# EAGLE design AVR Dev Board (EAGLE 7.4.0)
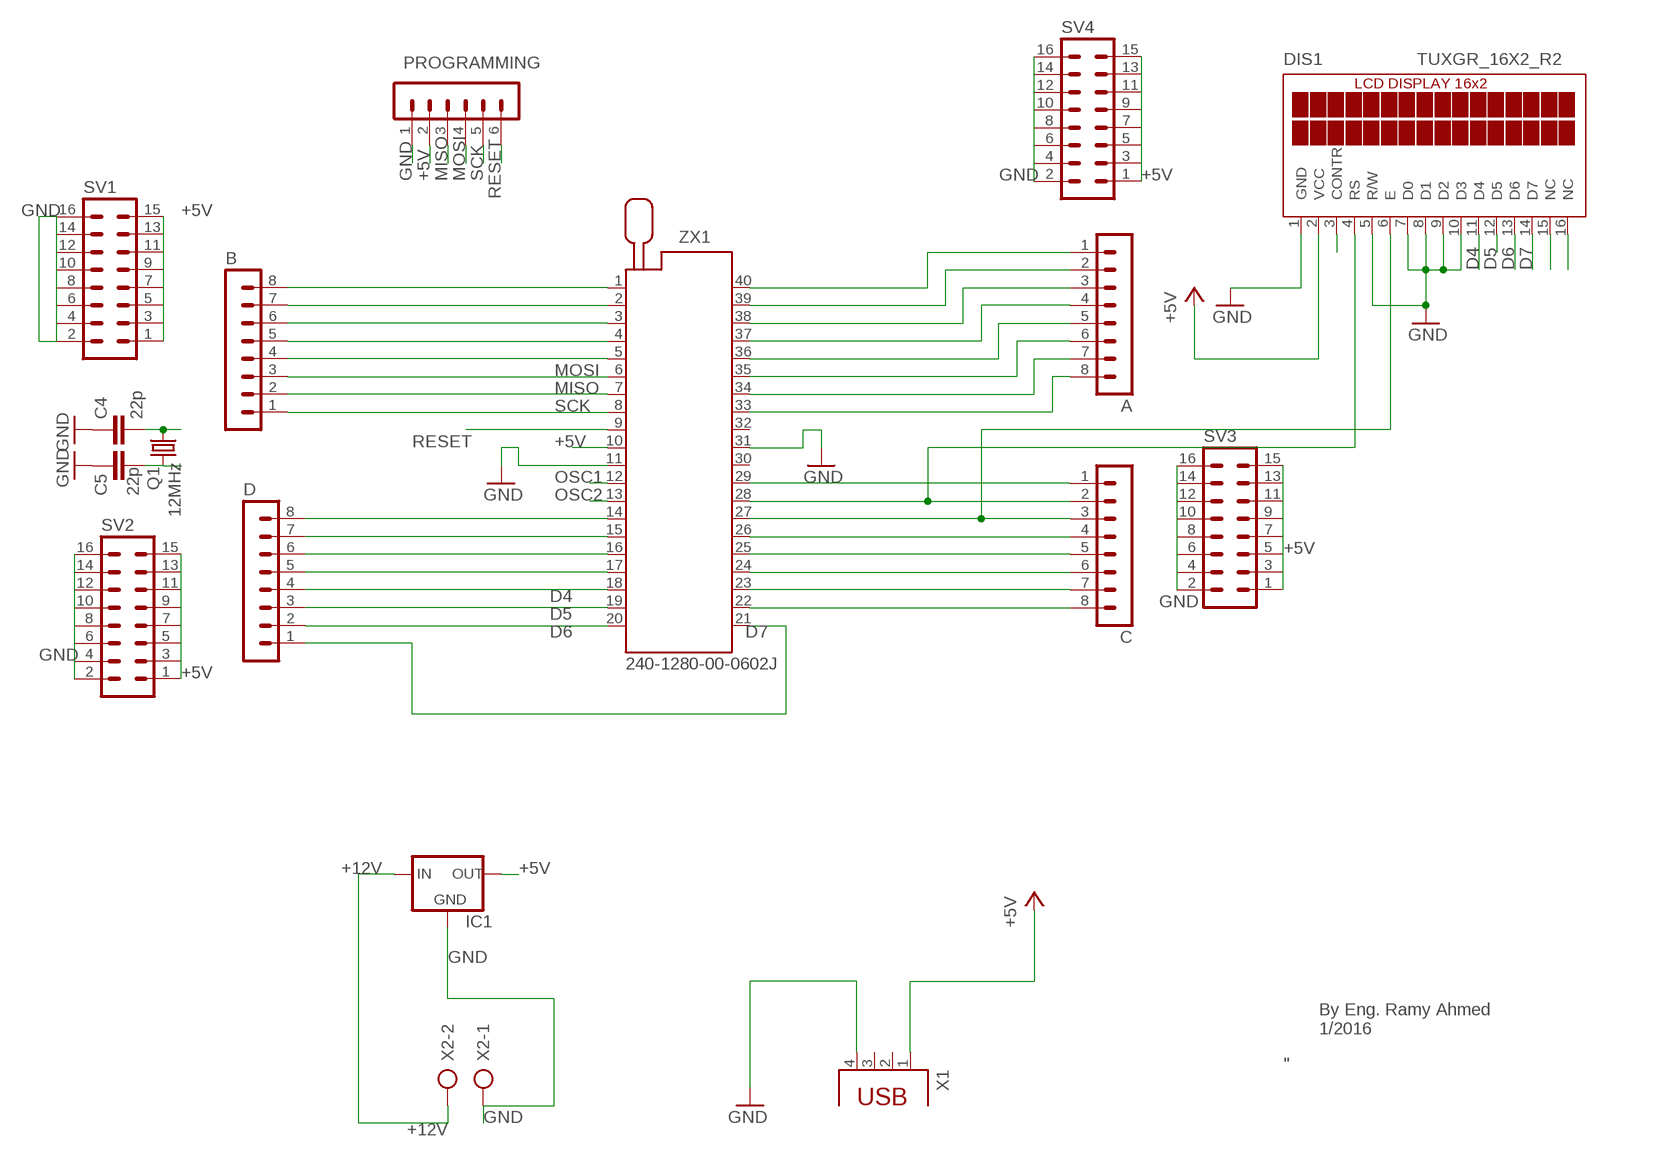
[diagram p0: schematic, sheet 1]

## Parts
A  MA08-1  [MA08-1]
B  MA08-1  [MA08-1]
C  MA08-1  [MA08-1]
C4  22p  C-EU025-024X044  [C025-024X044]
C5  22p  C-EU025-024X044  [C025-024X044]
D  MA08-1  [MA08-1]
DIS1  TUXGR_16X2_R2  [TUXGR_16X2_R2]
IC1  78XXL  [78XXL]
PROGRAMMING  MA06-1  [MA06-1]
Q1  12MHz  CRYTALHC49S  [HC49/S]
SV1  MA08-2  [MA08-2]
SV2  MA08-2  [MA08-2]
SV3  MA08-2  [MA08-2]
SV4  MA08-2  [MA08-2]
X1  PN61729  [PN61729]
X2  AK500/2  [AK500/2]
ZX1  240-1280-00-0602J  [240-1280-00-0602J]

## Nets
+5V: DIS1.2(VCC) IC1.OUT PROGRAMMING.2 SV1.1 SV1.3 SV1.5 SV1.7 SV1.9 SV1.11 SV1.13 SV1.15 SV2.1 SV2.3 SV2.5 SV2.7 SV2.9 SV2.11 SV2.13 SV2.15 SV3.1 SV3.3 SV3.5 SV3.7 SV3.9 SV3.11 SV3.13 SV3.15 SV4.1 SV4.3 SV4.5 SV4.7 SV4.9 SV4.11 SV4.13 SV4.15 X1.1 ZX1.10
+12V: IC1.IN X2.2
D4: D.4 DIS1.11(D4) ZX1.18
D5: D.3 DIS1.12(D5) ZX1.19
D6: D.2 DIS1.13(D6) ZX1.20
D7: D.1 DIS1.14(D7) ZX1.21
GND: C4.1 C5.1 DIS1.1(GND) DIS1.5(R/W) DIS1.7(D0) DIS1.8(D1) DIS1.9(D2) DIS1.10(D3) IC1.GND PROGRAMMING.1 SV1.2 SV1.4 SV1.6 SV1.8 SV1.10 SV1.12 SV1.14 SV1.16 SV2.2 SV2.4 SV2.6 SV2.8 SV2.10 SV2.12 SV2.14 SV2.16 SV3.2 SV3.4 SV3.6 SV3.8 SV3.10 SV3.12 SV3.14 SV3.16 SV4.2 SV4.4 SV4.6 SV4.8 SV4.10 SV4.12 SV4.14 SV4.16 X1.4 X2.1 ZX1.11 ZX1.31
MISO: B.2 PROGRAMMING.3 ZX1.7
MOSI: B.3 PROGRAMMING.4 ZX1.6
N$1: A.6 ZX1.35
N$2: A.1 ZX1.40
N$3: A.2 ZX1.39
N$4: A.3 ZX1.38
N$5: A.4 ZX1.37
N$6: A.5 ZX1.36
N$7: A.8 ZX1.33
N$8: A.7 ZX1.34
N$9: C.8 ZX1.22
N$10: C.7 ZX1.23
N$11: C.6 ZX1.24
N$16: C.5 ZX1.25
N$18: C.4 ZX1.26
N$21: C.1 ZX1.29
N$29: D.5 ZX1.17
N$30: D.6 ZX1.16
N$31: D.7 ZX1.15
N$32: D.8 ZX1.14
N$33: B.8 ZX1.1
N$34: B.7 ZX1.2
N$35: B.6 ZX1.3
N$36: B.5 ZX1.4
N$37: B.4 ZX1.5
N$38: DIS1.3(CONTR)
N$39: C.2 DIS1.4(RS) ZX1.28
N$50: DIS1.15(NC)
N$51: DIS1.16(NC)
N$52: C.3 DIS1.6(E) ZX1.27
OSC1: C4.2 Q1.2 ZX1.12
OSC2: C5.2 Q1.1 ZX1.13
RESET: PROGRAMMING.6 ZX1.9
SCK: B.1 PROGRAMMING.5 ZX1.8
Unconnected: X1.2 X1.3 ZX1.30 ZX1.32

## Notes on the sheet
- By Eng. Ramy Ahmed
  1/2016
- " اللهم انى اعوذ بك من علم لا ينفع "

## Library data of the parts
A B C D = con-lstb:MA08-1: PIN HEADER; OC_FARNELL: unknown; OC_NEWARK: unknown
C4 C5 = rcl:C-EU: CAPACITOR, European symbol
DIS1 = display-lcd:TUXGR_16X2_R2: Tuxgraphics LCD display 16x2 characters reflective, without background light Source: tuxgr_12x2_r2.pdf; OC_FARNELL: unknown; OC_NEWARK: unknown
IC1 = v-reg-2:78XXL: VOLTAGE REGULATOR
PROGRAMMING = con-lstb:MA06-1: PIN HEADER; OC_FARNELL: unknown; OC_NEWARK: unknown
Q1 = crystal:CRYTAL: CRYSTAL
SV1-SV4 = con-lstb:MA08-2: PIN HEADER; OC_FARNELL: unknown; OC_NEWARK: unknown
X1 = con-berg:PN61729: BERG USB connector
X2 = con-ptr500:AK500/2: CONNECTOR; OC_FARNELL: unknown; OC_NEWARK: unknown
ZX1 = con-3m:240-?-00-0602J: Zero Insertion Force Socked Source: http://www.3M.com/ehpd; MF: 3M; MPN: 240-1280-00-0602J; OC_FARNELL: 9897364; OC_NEWARK: 85K7848

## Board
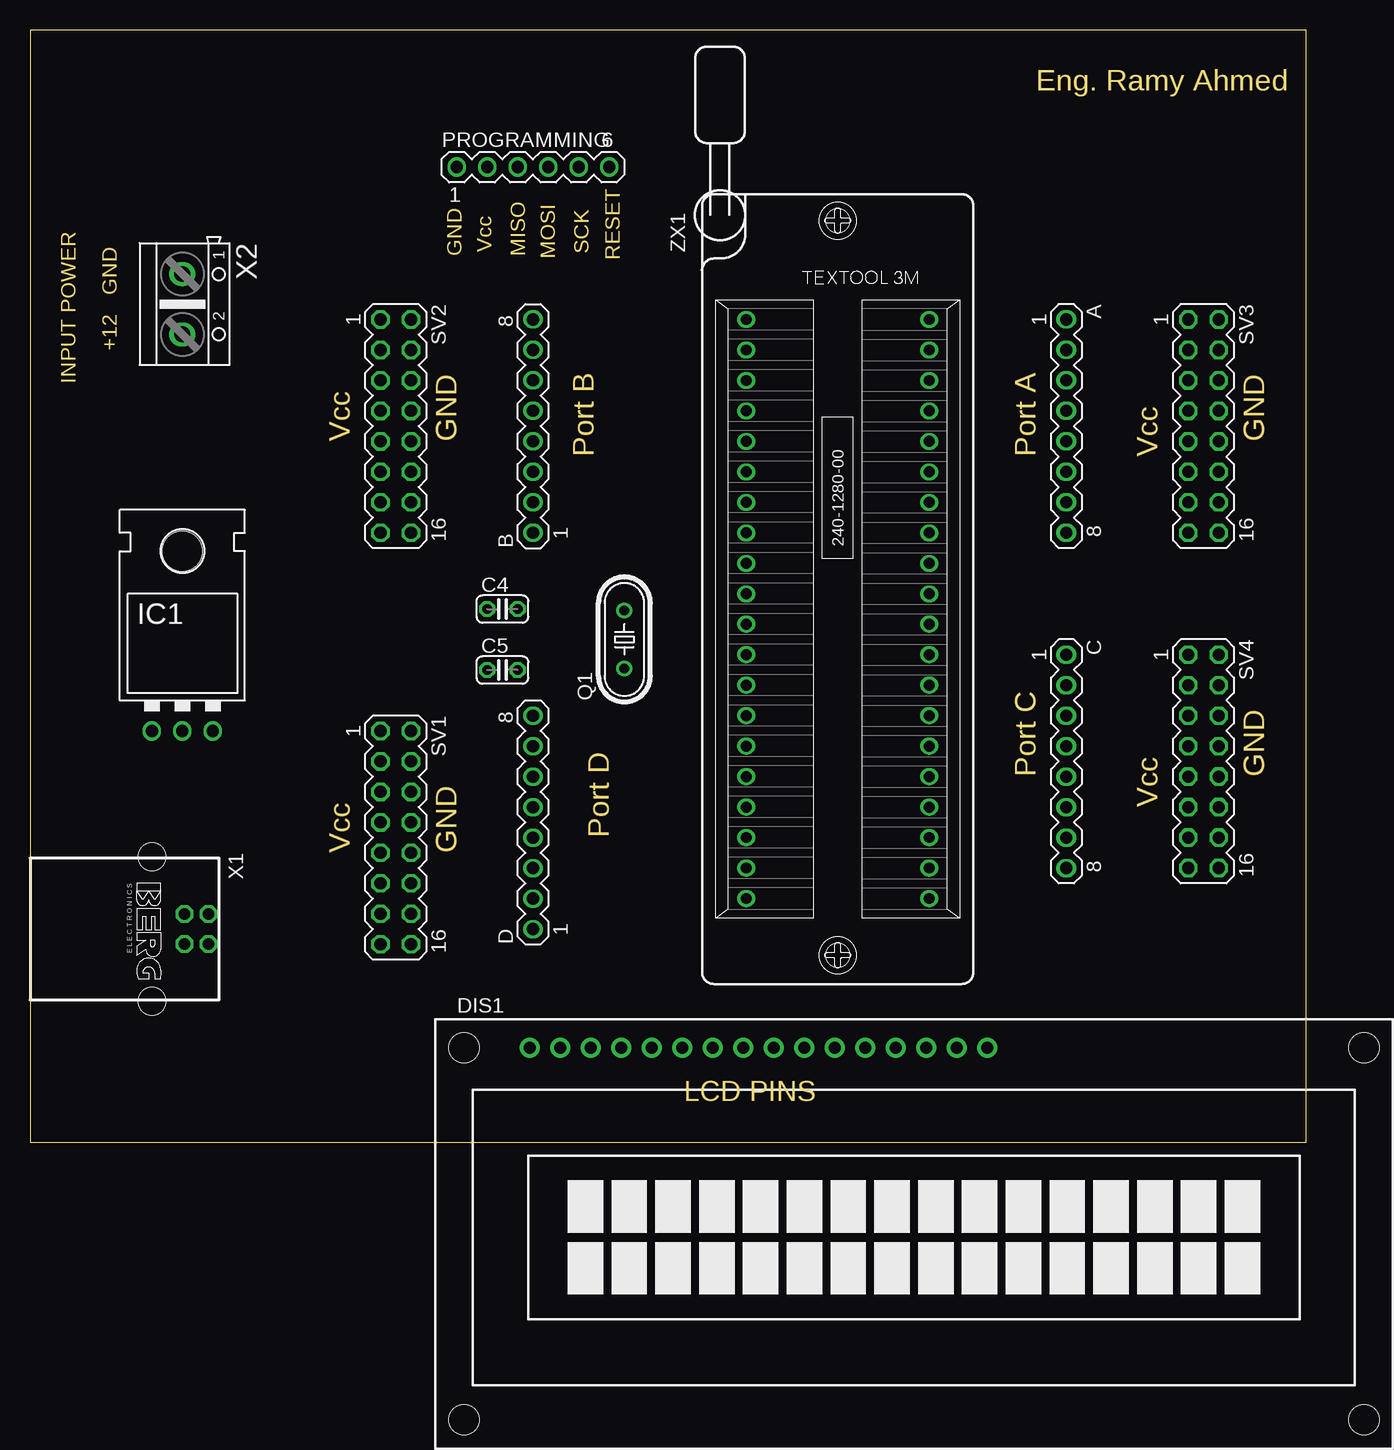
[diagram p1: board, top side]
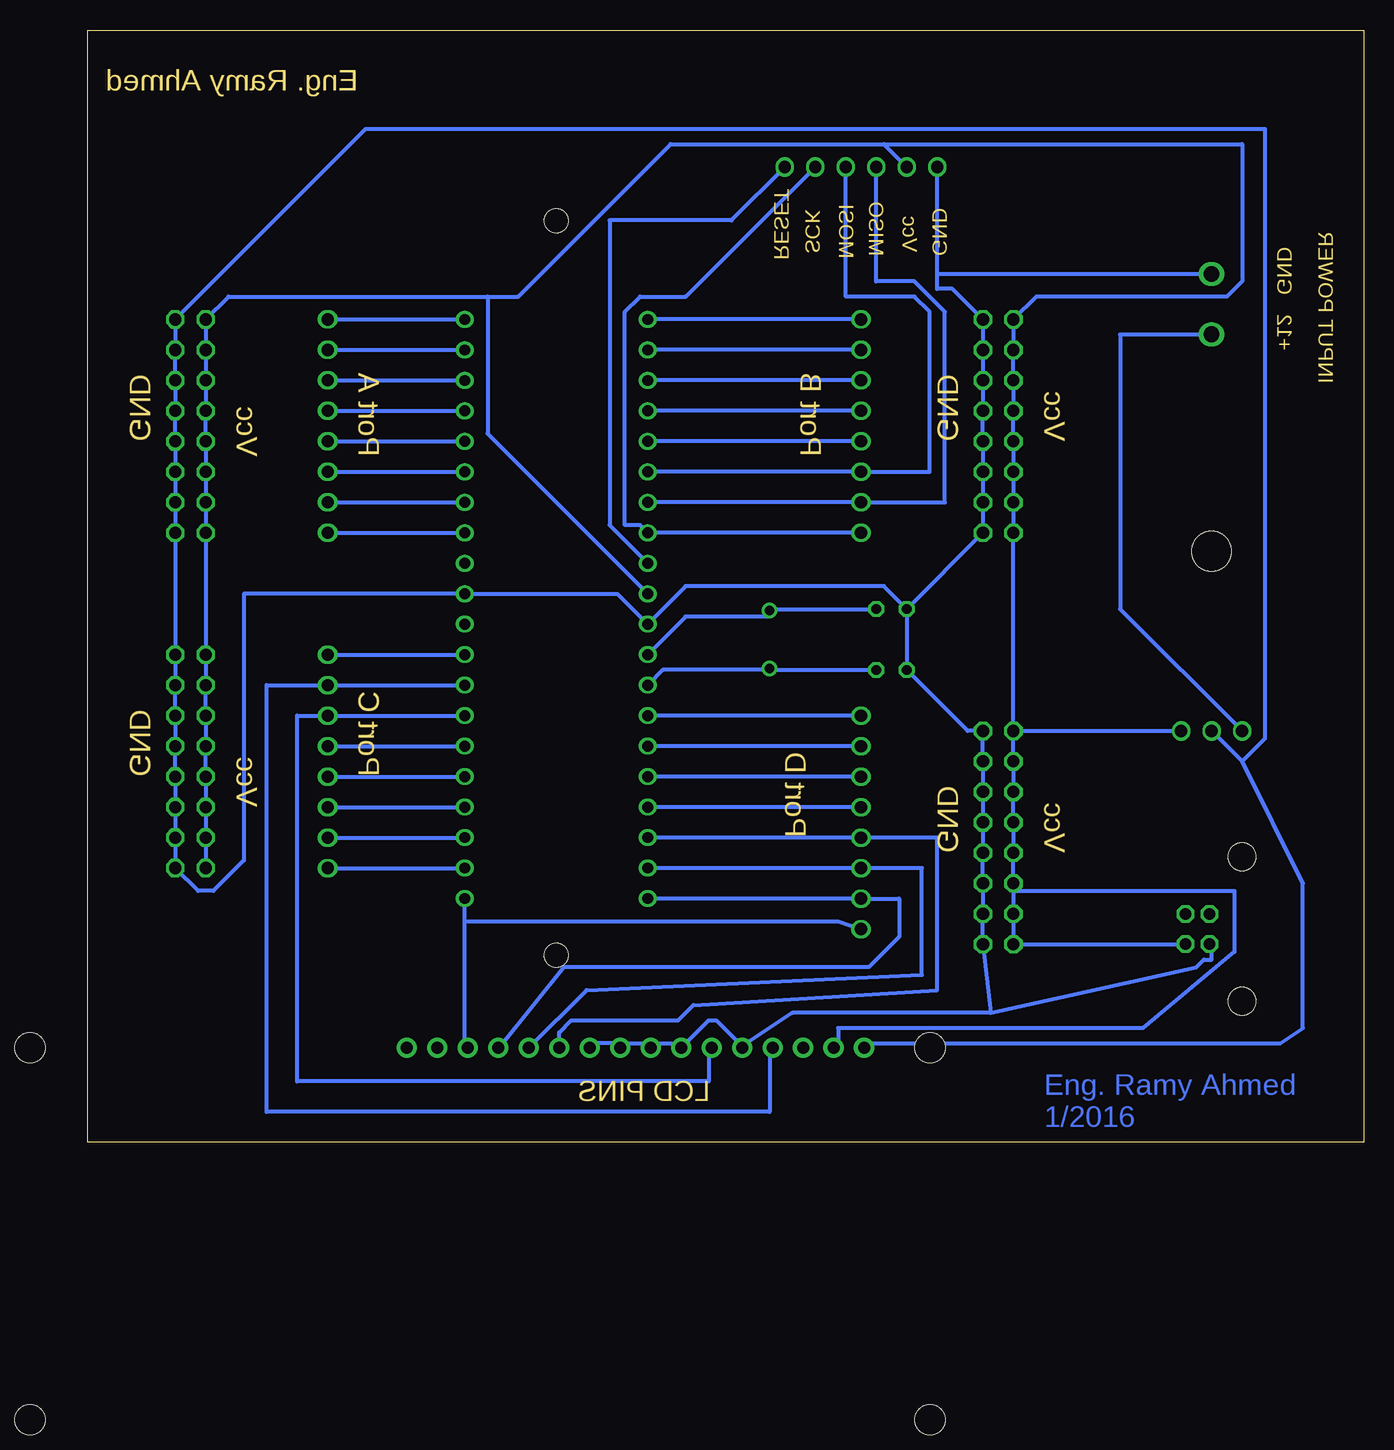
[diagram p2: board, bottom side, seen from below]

Size 106.35 x 92.7 mm. Coordinates in mm from the lower left corner, seen from the top.
Outline: 0,0 106.35,0 106.35,92.7 0,92.7 0,0
Copper layers (1*16): Top 0.035mm / dielectric 1.5mm / Bottom 0.035mm
Design rules "default *": minimum track width 0.35mm, minimum drill 0.6mm, track to track 0.5mm, track to pad 0.66mm, pad to pad 1mm, via to via 0.205mm, smd to smd 8mil, copper to edge 40mil, drill to drill 8mil, minimum pad ring 10mil, minimum via ring 8mil, stop-mask expansion 4mil, vias tented up to drill 0mil, thermal gap 10mil

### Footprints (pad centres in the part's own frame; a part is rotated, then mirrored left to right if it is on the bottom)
MA08-1 = drill 1.016 long: 1 -8.89,0; 2 -6.35,0; 3 -3.81,0; 4 -1.27,0; 5 1.27,0; 6 3.81,0; 7 6.35,0; 8 8.89,0
C025-024X044 = drill 0.813 octagon: 1 -1.27,0; 2 1.27,0
TUXGR_16X2_R2 = drill 1 pad 1.676: 1 -32,15.5; 2 -29.46,15.5; 3 -26.92,15.5; 4 -24.38,15.5; 5 -21.84,15.5; 6 -19.3,15.5; 7 -16.76,15.5; 8 -14.22,15.5; 9 -11.68,15.5; 10 -9.14,15.5; 11 -6.6,15.5; 12 -4.06,15.5; 13 -1.52,15.5; 14 1.02,15.5; 15 3.56,15.5; 16 6.1,15.5 | hole 2.5: -37.5,-15.5; 37.5,-15.5; -37.5,15.5; 37.5,15.5
78XXL = drill 1.016 long: GND 0,-3.81; IN -2.54,-3.81; OUT 2.54,-3.81 | hole 3.302: 0,11.176
MA06-1 = drill 1.016 long: 1 -6.35,0; 2 -3.81,0; 3 -1.27,0; 4 1.27,0; 5 3.81,0; 6 6.35,0
HC49/S = drill 0.813: 1 -2.413,0; 2 2.413,0
MA08-2 = drill 1.016 octagon: 1 -8.89,-1.27; 2 -8.89,1.27; 3 -6.35,-1.27; 4 -6.35,1.27; 5 -3.81,-1.27; 6 -3.81,1.27; 7 -1.27,-1.27; 8 -1.27,1.27; 9 1.27,-1.27; 10 1.27,1.27; 11 3.81,-1.27; 12 3.81,1.27; 13 6.35,-1.27; 14 6.35,1.27; 15 8.89,-1.27; 16 8.89,1.27
PN61729 = drill 0.95 octagon: 1 1.25,4.71; 2 -1.25,4.71; 3 -1.25,2.71; 4 1.25,2.71 | hole 2.3: -6.02,0; 6.02,0
AK500/2 = drill 1.321 long: 1 -2.515,0; 2 2.515,0
240-1280-00-0602J = drill 0.9 long: 1 -24.13,-7.62; 2 -21.59,-7.62; 3 -19.05,-7.62; 4 -16.51,-7.62; 5 -13.97,-7.62; 6 -11.43,-7.62; 7 -8.89,-7.62; 8 -6.35,-7.62; 9 -3.81,-7.62; 10 -1.27,-7.62; 11 1.27,-7.62; 12 3.81,-7.62; 13 6.35,-7.62; 14 8.89,-7.62; 15 11.43,-7.62; 16 13.97,-7.62; 17 16.51,-7.62; 18 19.05,-7.62; 19 21.59,-7.62; 20 24.13,-7.62; 21 24.13,7.62; 22 21.59,7.62; 23 19.05,7.62; 24 16.51,7.62; 25 13.97,7.62; 26 11.43,7.62; 27 8.89,7.62; 28 6.35,7.62; 29 3.81,7.62; 30 1.27,7.62; 31 -1.27,7.62; 32 -3.81,7.62; 33 -6.35,7.62; 34 -8.89,7.62; 35 -11.43,7.62; 36 -13.97,7.62; 37 -16.51,7.62; 38 -19.05,7.62; 39 -21.59,7.62; 40 -24.13,7.62 | hole 2: 28.86,0; -32.36,0

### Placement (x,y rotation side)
A  86.36,59.69 270 top
B  41.91,59.69 90 top
C  86.36,31.75 270 top
C4  39.37,44.45 0 top
C5  39.37,39.37 0 top
D  41.91,26.67 90 top
DIS1  73.66,-7.62 0 top
IC1  12.7,38.1 0 top
PROGRAMMING  41.91,81.28 0 top
Q1  49.53,41.91 90 top
SV1  30.48,25.4 270 top
SV2  30.48,59.69 270 top
SV3  97.79,59.69 270 top
SV4  97.79,31.75 270 top
X1  10.16,17.78 270 top
X2  12.7,69.85 270 top
ZX1  67.31,44.45 270 top

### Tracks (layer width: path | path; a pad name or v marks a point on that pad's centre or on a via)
+5V
  Bottom 0.35: X1.1 15.24,16.51 SV1.15 SV1.13 29.21,20.95 | SV1.1 IC1.OUT | 29.21,20.95 10.79,20.95 10.79,15.88 18.41,9.53 43.81,9.53 43.81,8.26 DIS1.2 | 29.21,20.95 SV1.11 SV1.9 SV1.7 SV1.5 SV1.3 SV1.1 | SV1.1 SV2.15 SV2.13 SV2.11 SV2.9 SV2.7 SV2.5 SV2.3 SV2.1 27.3,70.48 11.43,70.48 10.16,71.75 10.16,83.19 40.01,83.19 | SV4.15 SV4.13 SV4.11 SV4.9 SV4.7 SV4.5 SV4.3 SV4.1 SV3.15 SV3.13 SV3.11 SV3.9 SV3.7 SV3.5 SV3.3 SV3.1 94.61,70.48 73.03,70.48 | ZX1.10 73.03,59.05 73.03,70.48 | 40.01,83.19 PROGRAMMING.2 | 40.01,83.19 57.78,83.19 70.48,70.48 73.03,70.48
+12V
  Bottom 0.35: IC1.IN 20.32,44.45 20.32,67.31 12.7,67.31 X2.2
D4
  Bottom 0.35: ZX1.18 D.4 35.56,25.4 35.56,12.7 55.88,11.43 57.15,10.16 66.04,10.16 67.06,9.14 DIS1.11
D5
  Bottom 0.35: ZX1.19 43.18,22.86 D.3 36.83,22.86 36.83,13.97 64.77,12.7 DIS1.12
D6
  Bottom 0.35: ZX1.20 D.2 38.73,20.32 38.73,17.14 41.27,14.61 66.67,14.61 71.75,8.26 DIS1.13
D7
  Bottom 0.35: 74.93,18.41 74.93,8.26 DIS1.14 | 74.93,18.41 ZX1.21 | D.1 43.81,18.41 74.93,18.41
GND
  Bottom 0.35: DIS1.10 64.14,8.26 62.23,8.26 DIS1.9 61.59,8.26 59.69,8.26 DIS1.8 59.05,8.26 57.15,8.26 DIS1.7 56.52,8.26 54.61,10.16 53.98,10.16 52.07,8.26 DIS1.5 51.44,8.26 47.62,10.79 31.11,10.79 | 31.11,10.79 13.97,14.61 13.34,15.24 12.7,15.24 12.7,16.51 X1.4 | 31.11,10.79 SV1.16 SV1.14 SV1.12 SV1.10 SV1.8 SV1.6 SV1.4 SV1.2 33.02,34.29 C5.1 C4.1 | 10.16,31.75 5.08,21.59 5.08,9.53 6.99,8.26 41.27,8.26 DIS1.1 | 10.16,31.75 IC1.GND | 35.56,72.39 35.56,71.12 34.29,71.12 SV2.2 SV2.4 SV2.6 SV2.8 SV2.10 SV2.12 SV2.14 SV2.16 C4.1 | 35.56,72.39 PROGRAMMING.1 | 35.56,72.39 12.7,72.39 X2.1 | C4.1 40.01,46.35 56.52,46.35 ZX1.11 62.23,45.72 ZX1.31 93.34,45.72 93.34,23.5 95.89,20.95 97.16,20.95 SV4.16 SV4.14 SV4.12 SV4.10 SV4.8 SV4.6 SV4.4 SV4.2 SV3.16 SV3.14 SV3.12 SV3.10 SV3.8 SV3.6 SV3.4 SV3.2 83.19,84.45 8.26,84.45 8.26,33.66 10.16,31.75
MISO
  Bottom 0.35: ZX1.7 B.2 34.92,53.34 34.92,69.22 37.47,71.75 40.64,71.75 PROGRAMMING.3
MOSI
  Bottom 0.35: ZX1.6 B.3 36.2,55.88 36.2,69.22 37.47,70.48 43.18,70.48 PROGRAMMING.4
N$1
  Bottom 0.35: A.6 ZX1.35
N$2
  Bottom 0.35: A.1 ZX1.40
N$3
  Bottom 0.35: A.2 ZX1.39
N$4
  Bottom 0.35: A.3 ZX1.38
N$5
  Bottom 0.35: A.4 ZX1.37
N$6
  Bottom 0.35: A.5 ZX1.36
N$7
  Bottom 0.35: A.8 ZX1.33
N$8
  Bottom 0.35: A.7 ZX1.34
N$9
  Bottom 0.35: C.8 ZX1.22
N$10
  Bottom 0.35: C.7 ZX1.23
N$11
  Bottom 0.35: C.6 ZX1.24
N$16
  Bottom 0.35: C.5 ZX1.25
N$18
  Bottom 0.35: C.4 ZX1.26
N$21
  Bottom 0.35: C.1 ZX1.29
N$29
  Bottom 0.35: D.5 ZX1.17
N$30
  Bottom 0.35: D.6 ZX1.16
N$31
  Bottom 0.35: D.7 ZX1.15
N$32
  Bottom 0.35: D.8 ZX1.14
N$33
  Bottom 0.35: B.8 ZX1.1
N$34
  Bottom 0.35: B.7 ZX1.2
N$35
  Bottom 0.35: B.6 ZX1.3
N$36
  Bottom 0.35: B.5 ZX1.4
N$37
  Bottom 0.35: B.4 ZX1.5
N$39
  Bottom 0.35: ZX1.28 C.2 91.44,38.1 91.44,2.54 49.53,2.54 49.53,7.88 DIS1.4
N$52
  Bottom 0.35: ZX1.27 C.3 88.9,35.56 88.9,5.08 54.61,5.08 54.61,7.88 DIS1.6
OSC1
  Bottom 0.35: C4.2 49.53,44.45 Q1.2 49.53,43.81 56.52,43.81 ZX1.12
OSC2
  Bottom 0.35: 49.53,39.37 C5.2 | ZX1.13 58.42,39.37 49.53,39.37 | 49.53,39.37 Q1.1
RESET
  Bottom 0.35: ZX1.9 62.87,51.44 62.87,76.83 52.7,76.83 PROGRAMMING.6
SCK
  Bottom 0.35: B.1 ZX1.8 60.33,51.44 61.59,51.44 61.59,69.22 60.33,70.48 56.52,70.48 PROGRAMMING.5

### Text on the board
Bottom: Eng. Ramy Ahmed / 1/2016
Dimension: Eng. Ramy Ahmed | INPUT POWER | GND | GND | Vcc | MISO | MOSI | SCK | RESET | +12 | Vcc | GND | GND | Port B | Port A | Vcc | Port C | GND | Vcc | Port D | Vcc | GND | LCD PINS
